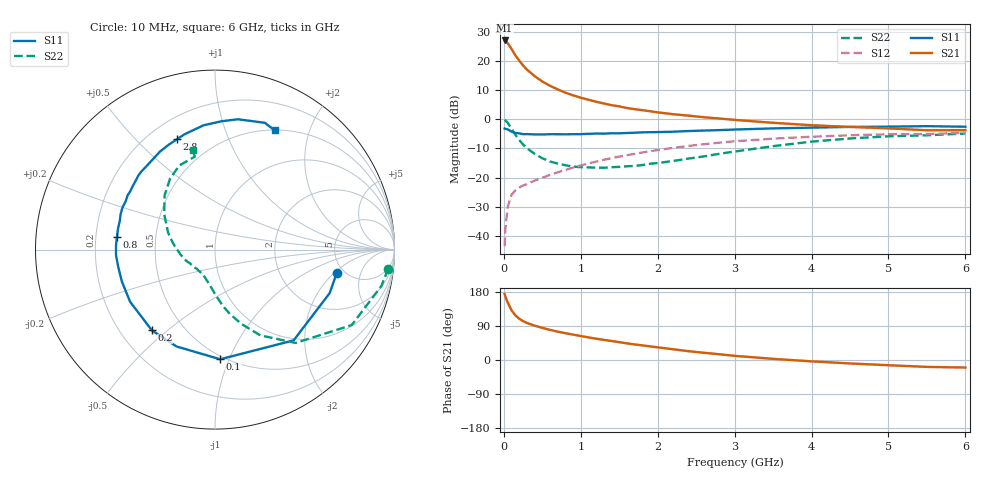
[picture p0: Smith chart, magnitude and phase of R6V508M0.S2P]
! SIEMENS Small Signal Semiconductors
! BFR193
! Si NPN RF Bipolar Junction Transistor in SOT23
! VCE = 0.5 V  IC = 8 mA
! Common Emitter S-Parameters:  May  1996
# GHz  S  MA  R  50
!  f  S11  S21  S12  S22
! GHz  MAG  ANG  MAG  ANG  MAG  ANG  MAG  ANG
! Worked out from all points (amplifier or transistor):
!   36 points, 10 MHz to 6 GHz, reference 50 ohm
!   highest |S21| = 27.0 dB at 10 MHz (marker M1)
!   |S21| within 3 dB of that: start of sweep to 102.2 MHz
!   unconditionally stable (mu >= 1): 717.5 MHz to 2.442 GHz
!   at 250 MHz: K = 0.60, MSG = 20.6 dB, |S12| = -22.7 dB
!   at 1.4 GHz: K = 1.07, MAG = 7.5 dB, |S12| = -13.3 dB
!   at 6 GHz: K = 1.00, MSG = 0.4 dB, |S12| = -4.6 dB
!   S11 on the Smith chart (normalised r, x): 10 MHz: 4.35, -2.16; 100 MHz: 0.48, -0.93; 200 MHz: 0.33, -0.44; 800 MHz: 0.29, +0.06; 2.8 GHz: 0.31, +0.66; 6 GHz: 0.50, +1.50
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0.01  0.6909 -10.8  22.26 174.1  0.0067 84.6  0.9714 -6.3
0.02  0.6833 -20.8  21.78 167.8  0.0134 79.1  0.9491 -12.3
0.05  0.6691 -49.1  20.04 151.5  0.0314 68.0  0.8701 -28.9
0.1  0.6116 -87.3  15.94 131.1  0.0507 54.9  0.687 -49.2
0.15  0.5807 -111.7  12.4 117.8  0.0606 48.3  0.5408 -62.1
0.2  0.5709 -128.1  10.05 109.1  0.0677 46.3  0.441 -70.3
0.25  0.5531 -139.9  8.31 102.5  0.0731 45.6  0.3678 -77.0
0.3  0.5552 -148.5  7.067 97.8  0.0778 46.5  0.3183 -81.9
0.4  0.5484 -161.2  5.463 90.7  0.0888 47.9  0.2551 -89.0
0.5  0.5477 -169.9  4.418 84.8  0.0995 49.9  0.2142 -95.3
0.6  0.5525 -177.0  3.729 79.5  0.1111 51.6  0.1888 -101.2
0.7  0.5521 177.4  3.235 74.8  0.123 52.7  0.1737 -106.3
0.8  0.551 172.5  2.848 70.8  0.1353 53.5  0.1626 -111.1
1.1  0.562 159.3  2.149 59.7  0.1745 54.0  0.1495 -124.5
1.3  0.5657 151.7  1.855 53.1  0.2019 53.2  0.1474 -134.1
1.6  0.5798 141.9  1.553 43.9  0.242 50.9  0.1562 -147.1
2.2  0.6103 124.7  1.216 28.3  0.3221 44.0  0.1924 -170.9
2.8  0.6499 109.1  1.027 15.2  0.3964 35.3  0.2553 165.7
3.5  0.6954 95.3  0.867 3.0  0.4641 24.1  0.3452 145.1
4.5  0.7371 80.1  0.737 -9.1  0.5305 9.7  0.4674 122.4
5.5  0.7591 68.5  0.646 -18.2  0.5554 -3.8  0.5298 102.3
6  0.743 63.5  0.648 -19.9  0.5866 -7.9  0.5677 102.4
